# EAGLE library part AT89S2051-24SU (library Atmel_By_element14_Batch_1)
8-bit Microcontroller with Flash
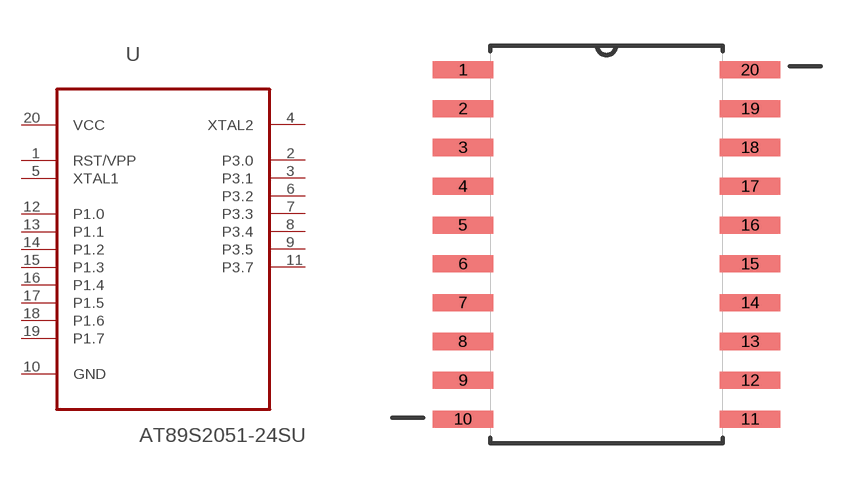
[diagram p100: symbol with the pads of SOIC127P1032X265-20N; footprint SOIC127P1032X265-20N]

Designator prefix U

## AT89S2051-24SU (MPN: AT89S2051-24SU; OC_FARNELL: 1095735; OC_NEWARK: 96K6574; PACKAGE: SOIC-20; SUPPLIER: Atmel)  [SOIC127P1032X265-20N]
1  RST/VPP  in
2  P3.0
3  P3.1
4  XTAL2  out
5  XTAL1
6  P3.2
7  P3.3
8  P3.4
9  P3.5
10  GND  pas
11  P3.7
12  P1.0
13  P1.1
14  P1.2
15  P1.3
16  P1.4
17  P1.5
18  P1.6
19  P1.7
20  VCC  pwr

## Footprint SOIC127P1032X265-20N (pad centres in mm)
smd 1.981 x 0.559: 1 -4.699,5.715; 2 -4.699,4.445; 3 -4.699,3.175; 4 -4.699,1.905; 5 -4.699,0.635; 6 -4.699,-0.635; 7 -4.699,-1.905; 8 -4.699,-3.175; 9 -4.699,-4.445; 10 -4.699,-5.715; 11 4.699,-5.715; 12 4.699,-4.445; 13 4.699,-3.175; 14 4.699,-1.905; 15 4.699,-0.635; 16 4.699,0.635; 17 4.699,1.905; 18 4.699,3.175; 19 4.699,4.445; 20 4.699,5.715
